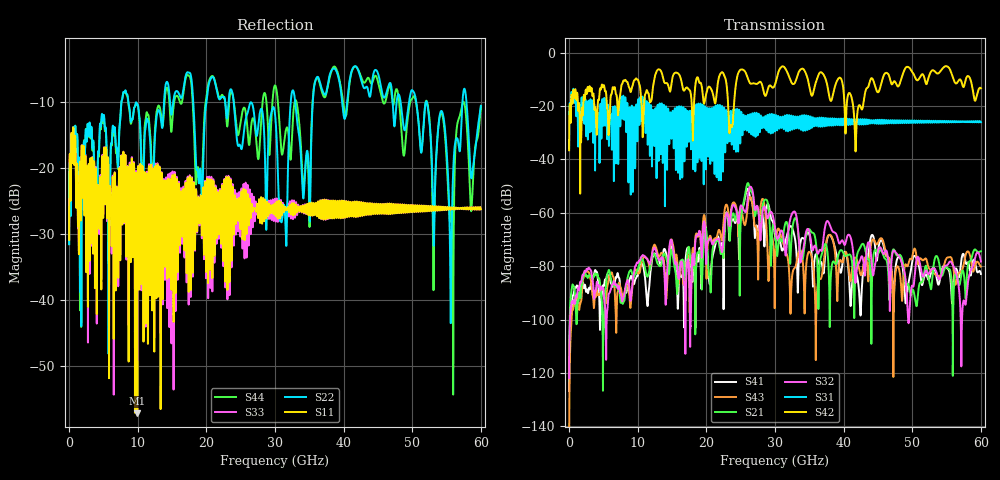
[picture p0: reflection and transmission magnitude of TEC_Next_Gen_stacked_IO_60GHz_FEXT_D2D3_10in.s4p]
!! CHANNEL DESCRIPTION:  Next Generation 28Gbps Press-fit Stacked I/O Connector
!!  with 10" 5-6-5 Megtron 6 Stripline trace on host side and 1.25" 7-5-7 Megtron 6 Microstrip trace on plug side
!! HOST PCB DESCRIPTION:  PCB thickness 3.425 mm
!!  26 Layer Board, 15 GND planes, 4 Layer route-out on Layers 7,11,17,21, 8mil stub on vias
!!  Pairs on following layers
!!  Layer 07 - A02A03 A14A15 D05D06
!!  Layer 11 - D020D3 C05C06 D14D15
!!  Layer 17 - C02C03 B05B06 C14C15
!!  Layer 21 - B02B03 A05A06 B14B15
!! CONNECTOR DESCRIPTION:  Next Generation 28Gbps Press-fit Stacked I/O Connector
!! PLUG-IN CARD DESCRIPTION:  PCB thickness 1mm thick
!!  6 Layer Board, 4 GND planes, 0.35 x 1.4mm mating pads
!!  Micro-strip diff traces referenced to GND plane 3mils down, 2nd GND plane 17mils from top of board
!!  PCB GND planes are symmetric
!! MODEL DESCRIPTION: TE Connectivity S-parameter model produced from Macro-model, Extracted .s4p FEXT (Victim B05B06 - Aggressor D02D03)
!! MODEL DATE: 5/15/2014 CR32f, FPR23
!! MODEL STATUS: Developmental
!! MODEL GEOMETRY: 4 Rows - Rows A, B, C, D. 3 pairs in each row, 12 total pairs
!! MODEL FREQUENCY RANGE: DC to 60 GHz in 10 MHz frequency steps
!! MODEL EDGE RATE LIMITATION: 8.33 ps (Using conservative 0.5/Fmax rule of thumb)
!! TIME-DOMAIN TRANSFORM CAUTIONS:
!! 1.) Do not simulate transient edge rates faster than the number listed above.  Edge
!!  rates faster than this number contain significant spectral content at frequencies
!!  above the model's highest frequency.
!! 2.) Even when simulating edge rates that are slower than the number listed above, be
!!  aware that the best time resolution possible with a direct iFFT is (1 / 2Fmax).
!!  As a result, time resolution is typically not adequate for most time-domain
!!  simulations unless tricks such as frequency-domain zero-padding and windowing are
!!  used to minimize leakage and aliasing.
!! 3.) Because the model has a uniform frequency step, a direct iFFT will result in an
!!  impulse that that has a time length given by either (1 / Fstep) or (1 / 2Fstep),
!!  depending on the transform being used.  Care has been taken in selecting the
!!  frequency step to ensure a settled impulse response for the model.  Therefore,
!!  convolution with the model's impulse response should present no issues.  However,
!!  if directly concatenating s-parameter models in the frequency domain a user must
!!  either interpolate necessary interim frequencies or complete impulse response
!!  zero-padding.  Impulse response zero-padding is more difficult, but more accurate.
!! PORT DEFINITIONS:
!! Port  1  ----->  Host D02		B05 Module <-----  Port  2
!! Port  3  ----->  Host D03		B06 Module <-----  Port  4
! Touchstone data
! Created: 29-Sep-2014 by IdEM R2011 (7.0.3)
# Hz S MA R 50
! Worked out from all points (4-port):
!   6000 points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, 10 MHz to 60 GHz, reference 50 ohm
!   strongest paths, dB at 10 MHz, 15.01 GHz, 30.01 GHz, 45.01 GHz, 60 GHz:
!     S42: -36.6, -10.1, -12.0, -14.9, -13.4
!     S31: -35.8, -25.1, -29.5, -25.4, -26.1
!     S32: -121.9, -71.4, -65.7, -74.3, -78.3
!     S21: -119.5, -74.5, -66.8, -75.3, -74.4
!     S43: -144.8, -70.5, -82.0, -71.2, -80.2
!     S41: -126.7, -72.7, -69.0, -74.7, -82.9
!   lowest |S11| = -57.2 dB at 9.93 GHz (marker M1), VSWR 1.00, Z = 49.9 + j0.0188 ohm
!   |S11| at or under -10 dB: start of sweep to end of sweep
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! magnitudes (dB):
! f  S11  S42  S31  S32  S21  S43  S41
! 10 MHz  -30.9  -36.6  -35.8  -121.9  -119.5  -144.8  -126.7
! 9.93 GHz  -57.2  -10.1  -29.6  -78.7  -81.6  -81.5  -83.6
! 26.07 GHz  -24.9  -9.8  -23.3  -53.4  -48.9  -56.8  -51.1
! 36.42 GHz  -27.4  -8.0  -24.9  -74.4  -84.2  -85.0  -79.3
! 41.76 GHz  -27.2  -36.1  -25.5  -85.7  -80.3  -76.9  -82.2
! 55.58 GHz  -26.4  -6.9  -25.6  -78.2  -82.3  -76.6  -85.1
! 60 GHz  -26.3  -13.4  -26.1  -78.3  -74.4  -80.2  -82.9
